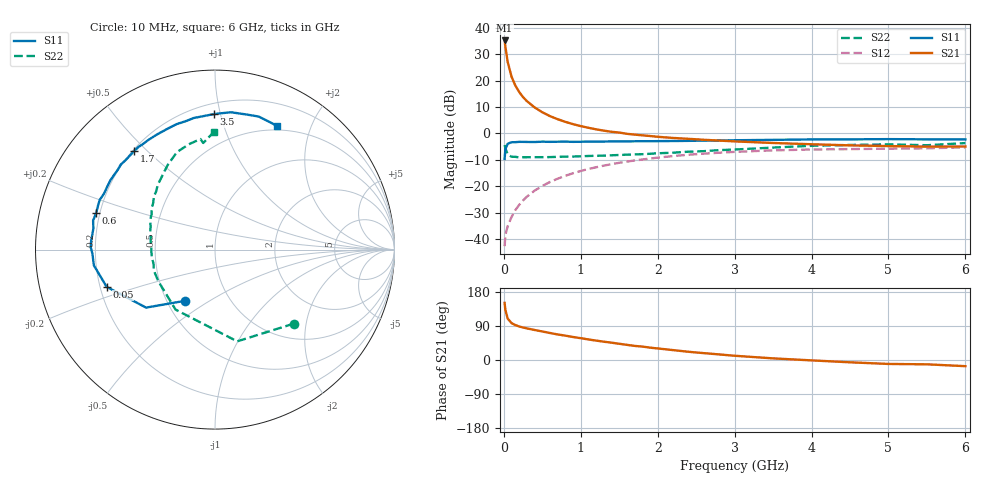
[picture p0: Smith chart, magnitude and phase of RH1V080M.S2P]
! SIEMENS Small Signal Semiconductors
! BFR106
! Si NPN RF Bipolar Junction Transistor in SOT23
! VCE = 1 V  IC = 80 mA
! Common Emitter S-Parameters:  August  1996
# GHz  S  MA  R  50
!  f  S11  S21  S12  S22
! GHz  MAG  ANG  MAG  ANG  MAG  ANG  MAG  ANG
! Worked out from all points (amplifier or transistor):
!   36 points, 10 MHz to 6 GHz, reference 50 ohm
!   highest |S21| = 35.2 dB at 10 MHz (marker M1)
!   |S21| within 3 dB of that: start of sweep to 23.45 MHz
!   unconditionally stable (mu >= 1): 90.72 MHz to end of sweep
!   at 250 MHz: K = 1.22, MAG = 16.8 dB, |S12| = -25.4 dB
!   at 1.4 GHz: K = 1.16, MAG = 3.7 dB, |S12| = -11.6 dB
!   at 6 GHz: K = 1.04, MAG = -1.0 dB, |S12| = -5.3 dB
!   S11 on the Smith chart (normalised r, x): 10 MHz: 0.62, -0.40; 50 MHz: 0.23, -0.16; 600 MHz: 0.19, +0.15; 1.7 GHz: 0.21, +0.46; 3.5 GHz: 0.27, +0.96; 6 GHz: 0.45, +1.53
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0.01  0.3288 -120.0  57.84 150.8  0.0073 64.5  0.6019 -43.3
0.02  0.5018 -139.9  44.22 132.2  0.0118 54.7  0.5259 -76.4
0.05  0.6382 -161.0  22.65 109.3  0.0175 53.2  0.4001 -123.3
0.1  0.6806 -172.6  11.92 97.4  0.0261 60.2  0.3616 -150.7
0.15  0.6833 -178.1  8.05 92.1  0.0353 65.2  0.3601 -161.1
0.2  0.6923 179.0  6.091 88.4  0.0443 68.1  0.3514 -166.9
0.25  0.6919 176.2  4.866 85.6  0.0536 69.6  0.3533 -171.5
0.3  0.6897 174.2  4.092 83.4  0.0634 70.8  0.3542 -173.9
0.4  0.6877 170.2  3.112 79.2  0.0824 71.0  0.3549 -178.3
0.5  0.6981 166.6  2.519 75.3  0.1011 70.3  0.3549 178.3
0.6  0.6927 162.9  2.126 71.2  0.1202 69.2  0.356 175.9
0.7  0.6963 159.3  1.861 67.4  0.1389 68.0  0.3603 173.6
0.8  0.6995 156.7  1.657 64.3  0.1575 66.1  0.3633 171.1
0.9  0.6925 153.2  1.5 60.7  0.1762 64.6  0.3647 168.6
1.1  0.6992 146.5  1.279 54.2  0.2117 60.9  0.374 165.0
1.3  0.7008 140.7  1.13 48.3  0.2454 56.9  0.3803 160.6
1.7  0.7105 129.4  0.95 37.2  0.307 49.3  0.4012 152.8
2.2  0.7181 116.9  0.821 26.1  0.3723 39.7  0.4313 143.0
3.5  0.7553 90.4  0.659 4.3  0.4777 17.6  0.5397 119.3
4.5  0.7725 77.2  0.594 -6.1  0.5051 4.1  0.6048 103.9
5.5  0.7733 66.8  0.563 -11.4  0.523 -3.6  0.5975 96.3
6  0.7704 63.3  0.566 -16.3  0.5445 -9.9  0.6569 90.4
